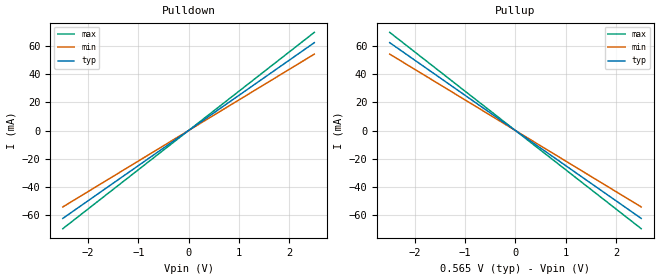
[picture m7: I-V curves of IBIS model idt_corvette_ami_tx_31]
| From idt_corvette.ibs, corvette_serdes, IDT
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|   model   idt_corvette_ami_tx_31
[Model] idt_corvette_ami_tx_31
Model_type Output
C_comp 400f 400f 400f
Cref = 0
[Model Spec]
Vmeas 0. 0. 0.
Vref 0. 0. 0.
[Temperature Range]  25 100 0
[Voltage Range] .565 .59 .475
[Algorithmic Model]
Executable Windows_VisualStudio5_32 idt_corvette_tx.dll   idt_corvette_tx.ami
Executable Windows_ver_64   idt_corvette_tx_64.dll   idt_corvette_tx.ami
Executable Linux_gcc4.1.2_32   idt_corvette_tx.linux.so   idt_corvette_tx.ami
Executable Linux_gcc3.2.3_64   idt_corvette_tx_64.linux.so idt_corvette_tx.ami
[End Algorithmic Model]
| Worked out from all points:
|   slope of the pulldown table from 0 to 0.085 V, typ, clamps not added: 40 ohm
|   slope of the pullup table from 0 to 0.085 V, typ, clamps not added: 40 ohm
[Pulldown]
-2.5V     -62.5mA    -54.35mA   -69.81mA
0V        0A         0A         0A
2.5V      62.5mA     54.35mA    69.81mA
[Pullup]
-2.5V     62.5mA     54.35mA    69.81mA
0V        0A         0A         0A
2.5V      -62.5mA    -54.35mA   -69.81mA
[Ramp]
dV/dt_r .188/22.4p .184/25.76p .166/20.054p
dV/dt_f .188/22.4p .184/25.76p .166/20.054p
